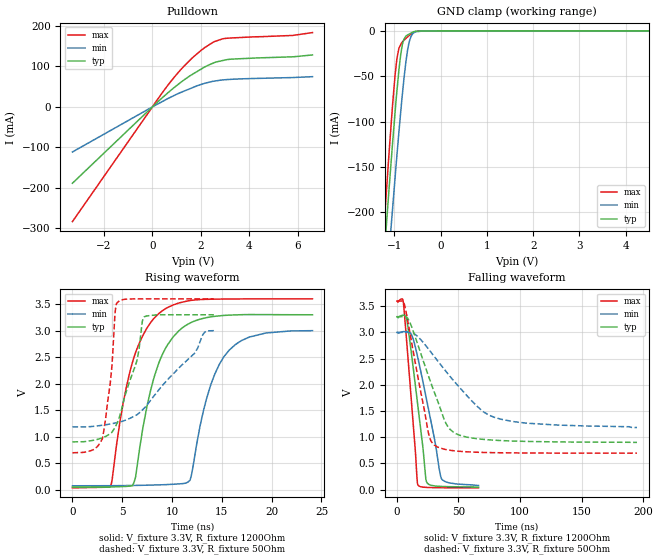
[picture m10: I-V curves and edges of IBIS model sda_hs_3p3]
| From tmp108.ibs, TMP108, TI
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|   sda_hs_3p3 Model
[Model]   sda_hs_3p3
Model_type   I/O_open_drain
Polarity   Non-Inverting
Vinl = 0.5
Vinh = 1.4
Vmeas = 1.65
Vref = 3.3
Cref = 2pF
Rref = 1200
|   typ   min   max
C_comp   6.770e-13   6.770e-13   7.186e-13
| Where nom  PVT is Nominal Process, 3.3V, 27C
|   Fast PVT is Strong Process,  3.6V, -40C
|   Slow PVT is Weak Process,   3V, 125C
[Voltage Range]   3.3   3   3.6
|Ambient Temperature   25   125   -40
|Junction Temperature
[Temperature Range]   27   125   -40
[Pullup Reference]   3.3   3   3.6
[Pulldown Reference]   0   0   0
[Power Clamp Reference]   3.3   3   3.6
[GND Clamp Reference]   0   0   0
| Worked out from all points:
|   slope of the pulldown table from 0 to 0.495 V, typ, clamps not added: 18.2 ohm
|   GND clamp passes 1 mA (typ) near -0.58 V on its own axis
|   falling waveform, V_fixture 3.3V, R_fixture 1200Ohm: 20-80 % time 10.1ns typ, 14.7ns min, 7.22ns max; typ from 3.3 V to 0.048 V
|   rising waveform, V_fixture 3.3V, R_fixture 1200Ohm: 20-80 % time 2.61ns typ, 2.61ns min, 2.65ns max; typ from 0.048 V to 3.3 V
|   falling waveform, V_fixture 3.3V, R_fixture 50Ohm: 20-80 % time 21.5ns typ, 40ns min, 13.7ns max; typ from 3.3 V to 0.901 V
|   rising waveform, V_fixture 3.3V, R_fixture 50Ohm: 20-80 % time 2.07ns typ, 5.22ns min, 897ps max; typ from 0.901 V to 3.3 V
[Pulldown]
|   Voltage   I(typ)   I(min)   I(max)
-3.3V     -188.7mA   -111.5mA   -283.5mA
633mV     34.54mA    20.43mA    53.27mA
1.246V    63.96mA    37.48mA    97.08mA
1.598V    78.58mA    46.12mA    118.4mA
2.012V    93.43mA    55.43mA    139.8mA
2.549V    109.1mA    63.56mA    161.1mA
2.934V    114.9mA    66.72mA    168.4mA
3.241V    117.9mA    67.98mA    170.2mA
5.774V    123.6mA    72.4mA     176.4mA
6.6V      128.3mA    74.58mA    183.5mA
[GND Clamp]
|   Voltage   I(typ)   I(min)   I(max)
-3.3V     -1.734A    -1.745A    -1.76A
-1.247V   -268.6mA   -335mA     -237mA
-1.119V   -179.7mA   -249.4mA   -140.5mA
-1.105V   -170.3mA   -240.6mA   -130.3mA
-1.037V   -124.9mA   -197.3mA   -82.91mA
-979.2mV  -88.9mA    -160.8mA   -48.16mA
-939.6mV  -65.66mA   -136.4mA   -30.04mA
-858mV    -25.6mA    -88.66mA   -15.11mA
-792mV    -9.495mA   -54.13mA   -10.6mA
-711mV    -4.601mA   -21.31mA   -6.699mA
-590.7mV  -1.091mA   -2.61mA    -2.149mA
6.6V      0A         0A         0A
[POWER Clamp]
|   Voltage   I(typ)   I(min)   I(max)
-3.3V     0A         0A         0A
-3.298V   0A         0A         0A
6.6V      0A         0A         0A
[Ramp]
R_load = 1200
|   typ   min   max
dV/dt_r   1.95148/2.60733e-09   1.75647/2.59553e-09   2.13997/2.65576e-09
dV/dt_f   1.95148/1.00551e-08   1.75647/1.47565e-08   2.13997/7.21898e-09
[Falling Waveform]
V_fixture = 3.3V
V_fixture_min = 3V
V_fixture_max = 3.6V
R_fixture = 1200Ohm
|   Time   V(typ)   V(min)   V(max)
0s        3.3V       3V         3.6V
4.34ns    3.325V     3.012V     3.641V
5.27ns    3.328V     3.015V     3.562V
8.05ns    3.237V     3.016V     2.79V
12.05ns   2.548V     2.948V     1.604V
16.86ns   1.626V     2.53V      100.5mV
20.94ns   837.8mV    2.079V     47.58mV
23.9ns    159.1mV    1.739V     42.3mV
36.06ns   60.92mV    214.8mV    36.19mV
66.27ns   48.35mV    77.58mV    33.52mV
[Rising Waveform]
V_fixture = 3.3V
V_fixture_min = 3V
V_fixture_max = 3.6V
R_fixture = 1200Ohm
|   Time   V(typ)   V(min)   V(max)
0s        47.53mV    72.55mV    33.38mV
3.79ns    50.35mV    73.77mV    46.57mV
5.08ns    58mV       76.13mV    1.62V
6.02ns    74.99mV    78.4mV     2.4V
7.58ns    1.656V     84.03mV    3.079V
8.81ns    2.457V     90.47mV    3.345V
11.81ns   3.144V     177.4mV    3.568V
13.47ns   3.246V     1.72V      3.591V
15.74ns   3.293V     2.632V     3.598V
24.1ns    3.3V       3V         3.6V
[Falling Waveform]
V_fixture = 3.3V
V_fixture_min = 3V
V_fixture_max = 3.6V
R_fixture = 50Ohm
|   Time   V(typ)   V(min)   V(max)
0s        3.3V       3V         3.6V
6.38ns    3.301V     3.001V     3.508V
11.6ns    3.129V     2.996V     2.855V
25.75ns   2.16V      2.68V      1.066V
30.37ns   1.859V     2.54V      849.6mV
39.34ns   1.289V     2.271V     766.9mV
46.1ns    1.092V     2.078V     741.8mV
65.21ns   971.3mV    1.59V      713.1mV
78.46ns   944.1mV    1.385V     705.4mV
195ns     901.2mV    1.184V     695.2mV
[Rising Waveform]
V_fixture = 3.3V
V_fixture_min = 3V
V_fixture_max = 3.6V
R_fixture = 50Ohm
|   Time   V(typ)   V(min)   V(max)
0s        901.2mV    1.184V     695.2mV
3ns       976.4mV    1.215V     956.9mV
3.78ns    1.054V     1.238V     1.983V
4.27ns    1.175V     1.256V     3.309V
4.48ns    1.254V     1.265V     3.527V
6.47ns    2.43V      1.413V     3.6V
7.2ns     3.26V      1.537V     3.6V
12.26ns   3.3V       2.574V     3.6V
13.29ns   3.3V       2.972V     3.6V
14.2ns    3.3V       3V         3.6V
